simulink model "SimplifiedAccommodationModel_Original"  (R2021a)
settings: Solver=VariableStepAuto  StartTime=0.0  StopTime=10  FixedStep=0.00005  RelTol=1e-3  EnableMultiTasking=on
model workspace (MAT data in the model file):
  AccomRange : Simulink.Parameter (value not decoded)
  FastIntegGain : Simulink.Parameter (value not decoded)
  FastIntegTimeConstant : Simulink.Parameter (value not decoded)
  MinAccomSignal = 0.2
  MotorLatency : Simulink.Parameter (value not decoded)
  NeuralBias : Simulink.Parameter (value not decoded)
  PlantTimeConstant : Simulink.Parameter (value not decoded)
  RefractiveError : Simulink.Parameter (value not decoded)
  SensoryLatency : Simulink.Parameter (value not decoded)
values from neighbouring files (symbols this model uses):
  AccomRange = 6    [PlotSignalsForHyperopePlusLens.m]    (also in PlotACAratio.m = 2; PlotACAratioCycloplegia.m = 10; PlotACAratioCycloplegiaPresbyope.m = 1; PlotNearpointCycloplegia.m = 10)
  NeuralBias = getVariable(workspace,'NeuralBias')    [PlotNearpointCycloplegia.m]    (also in PlotSignalsForMyope.m; PlotOcularPowerCycloplegia.m)
  RefractiveError = 0    [PlotSignalsForEmmetropePlusLens.m]    (also in PlotSignalsForMyope.m = 2)
symbols that are objects in the model workspace (value not decoded): FastIntegGain, FastIntegTimeConstant, MotorLatency, PlantTimeConstant, SensoryLatency

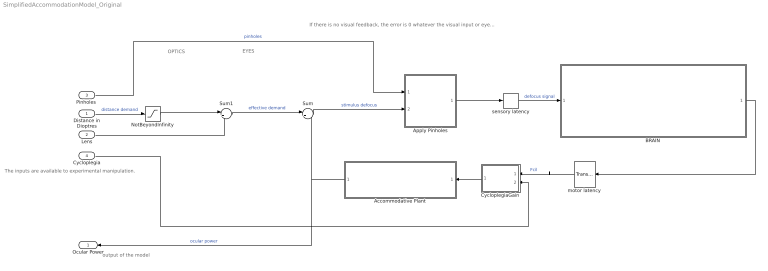
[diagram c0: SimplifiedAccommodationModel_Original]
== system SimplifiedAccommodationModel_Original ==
  note: output of the model
  note: The inputs are available to experimental manipulation.
  note: OPTICS
  note: EYES
  note: If there is no visual feedback, the error is 0 whatever the visual input or eye state
  Distance in Dioptres : Inport
  Lens : Inport  Port=2
  "Pinholes " : Inport  Port=3
  Cycloplegia : Inport  Port=4
  Accommodative Plant : Subsystem
  Apply Pinholes : MATLAB Function  TreatAsAtomicUnit=on
  BRAIN : Subsystem  Description=|
      | Accommodation system. 
      | It receives 3 inputs:
      | 1) Accommodative demand
      | 2) Convergence accommodation tonic signal
      | 3) Convergence accommodation phasic signal
      | 
      | It provides 3 outputs:
      | 1) The accommodation of the lens
      | 2) Accommodative convergence tonic signal
      | 2) Accommodative convergence phasic signal
  CycloplegiaGain : MATLAB Function  TreatAsAtomicUnit=on
  NotBeyondInfinity : Saturate  UpperLimit=100  LowerLimit=0
  Sum : Sum  Inputs=|+-  InputSameDT=on  SaturateOnIntegerOverflow=on
  Sum1 : Sum  Inputs=|+-
  motor latency : TransportDelay  DelayTime=MotorLatency
  sensory latency : TransportDelay  DelayTime=SensoryLatency
  Ocular Power : Outport
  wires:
  Distance in Dioptres/1 -> NotBeyondInfinity/1  "distance demand"
  Sum/1 -> Apply Pinholes/2(demand)  "stimulus defocus"
  Lens/1 -> Sum1/2
  Sum1/1 -> Sum/1  "effective demand"
  "Pinholes "/1 -> Apply Pinholes/1(pinholesON)  "pinholes"
  NotBeyondInfinity/1 -> Sum1/1
  Accommodative Plant/1(Ocular power) -> Sum/2, Ocular Power/1  "ocular power"
  Apply Pinholes/1(y) -> sensory latency/1
  sensory latency/1 -> BRAIN/1(Retinal defocus)  "defocus signal"
  motor latency/1 -> CycloplegiaGain/1(signal)  "Fcil"
  CycloplegiaGain/1(output) -> Accommodative Plant/1(Ciliary muscle input)
  Cycloplegia/1 -> CycloplegiaGain/2(drug)
  BRAIN/1(Oculomotor nerve signal) -> motor latency/1

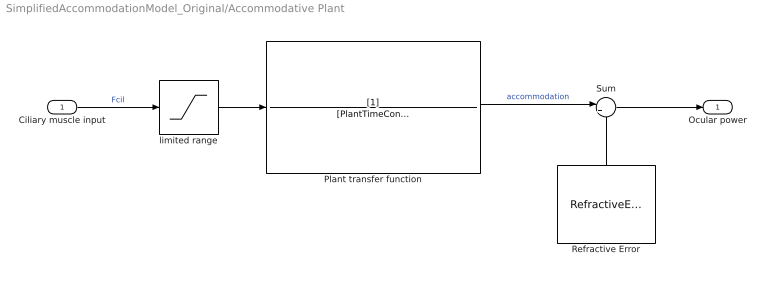
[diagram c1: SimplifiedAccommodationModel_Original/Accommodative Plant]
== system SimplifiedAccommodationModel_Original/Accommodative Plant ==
  Ciliary muscle input : Inport
  Plant transfer function : TransferFcn  Denominator=[PlantTimeConstant 1]
  Refractive Error : Constant  Value=RefractiveError
  Sum : Sum  Inputs=|++
  limited range : Saturate  UpperLimit=AccomRange  LowerLimit=0
  Ocular power : Outport
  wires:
  Ciliary muscle input/1 -> limited range/1  "Fcil"
  Refractive Error/1 -> Sum/2
  Sum/1 -> Ocular power/1
  Plant transfer function/1 -> Sum/1  "accommodation"
  limited range/1 -> Plant transfer function/1

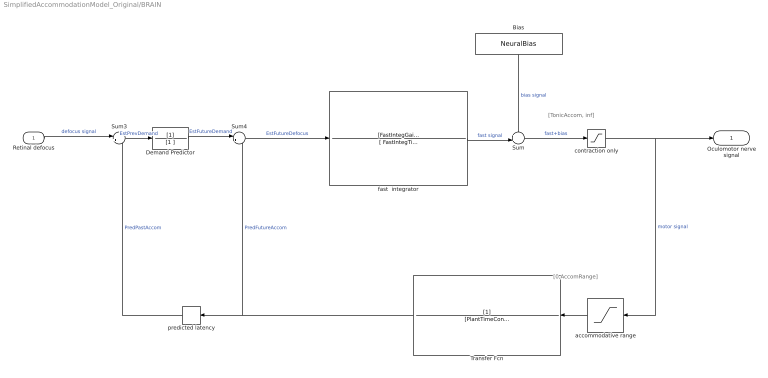
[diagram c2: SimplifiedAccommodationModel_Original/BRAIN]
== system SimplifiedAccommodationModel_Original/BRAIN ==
  note: [TonicAccom, inf]
  note: [0,AccomRange]
  Retinal defocus : Inport
  Bias : Constant  Value=NeuralBias
  Demand Predictor : TransferFcn  Denominator=[1 ]
  Sum : Sum  Inputs=++|
  Sum3 : Sum  Inputs=|++
  Sum4 : Sum  Inputs=|+-
  Transfer Fcn : TransferFcn  Denominator=[PlantTimeConstant 1]
  accommodative range : Saturate  UpperLimit=AccomRange  LowerLimit=0
  contraction only : Saturate  UpperLimit=Inf  LowerLimit=MinAccomSignal
  fast  integrator : TransferFcn  Numerator=[FastIntegGain]  Denominator=[ FastIntegTimeConstant 1]
  predicted latency : TransportDelay  DelayTime=SensoryLatency+MotorLatency
  Oculomotor nerve signal : Outport
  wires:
  Sum3/1 -> Demand Predictor/1  "EstPrevDemand"
  predicted latency/1 -> Sum3/2  "PredPastAccom"
  Sum4/1 -> fast  integrator/1  "EstFutureDefocus"
  Retinal defocus/1 -> Sum3/1  "defocus signal"
  contraction only/1 -> accommodative range/1, Oculomotor nerve signal/1  "motor signal"
  Transfer Fcn/1 -> Sum4/2, predicted latency/1  "PredFutureAccom"
  Bias/1 -> Sum/1  "bias signal"
  fast  integrator/1 -> Sum/2  "fast signal"
  Sum/1 -> contraction only/1  "fast+bias"
  Demand Predictor/1 -> Sum4/1  "EstFutureDemand"
  accommodative range/1 -> Transfer Fcn/1

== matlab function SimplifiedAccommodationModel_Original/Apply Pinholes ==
function y = fcn(pinholesON,demand)
if pinholesON>0
    y = 0;
else
    y = demand;
end

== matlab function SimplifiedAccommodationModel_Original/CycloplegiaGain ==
function output = fcn(signal,drug)
% Modeling cycloplegia as a gain

% Clip strength of drug to the range 0 to 1:
drug(drug<0) = 0;
drug(drug>1) = 1;
output = (1-drug)*signal;
